PROGRAM Auto
VAR
	//////////////////////自动////////////////////////////////////////////
	//输入
	start AT%I* : BOOL;                        //启动按钮
	stop AT%I* : BOOL;                         //停止按钮
	//延时
	delayed_time: TON;                         //下限位延时功能块
	//其他
	state:INT;                                 //状态
	R_TRIG: R_TRIG;                            //检测下限位上升沿信号
	cycle_count:INT;                           //计数
	//超时监控
	watch_timer :ARRAY[1..2]OF TON;//工作计时
	bErr: BOOL;//报错
	ierrorID: INT:=0;//报错代码
END_VAR

CASE state OF
	0://初始状态
	   solenoid_valve_up := FALSE;                                     //上行电磁阀松开
       solenoid_valve_down := FALSE;	                               //下行电磁阀松开
       cycle_count := 0;                                               // 重置循环次数
	   bErr :=FALSE;                                               //报错复位
	   ierrorID :=0;                                               //报错代码复位
	   IF start THEN
	      solenoid_valve_down := TRUE;                                 // 下行电磁阀吸合，气缸下行
          state := 1;                                              
	   END_IF
	1://下行阶段  
	  solenoid_valve_down := TRUE;
      IF limit_switch_down THEN                                      //到达下限位
         solenoid_valve_down := FALSE;                              //下行电磁阀松开
      END_IF;
		 delayed_time(IN:=limit_switch_down , PT:=T#3S , Q=> , ET=> );  // 启动3秒延时
      IF delayed_time.Q THEN
         solenoid_valve_up := TRUE;                                 // 上行电磁阀吸合
         state := 2;                                                                                                                   
      END_IF;
    2://上行阶段
	  solenoid_valve_up := TRUE;
	  R_TRIG(CLK:=limit_switch_UP , Q=> );
      IF R_TRIG.Q THEN
         cycle_count := cycle_count + 1;                              // 循环次数+1
         solenoid_valve_up := FALSE;                                  // 上行电磁阀松开
         state := 1;                                                  // 切换回下行状态（开始下一次循环）
      END_IF;
      IF cycle_count >= 3 THEN                                        //清洗次数达到3次回到初始位
         state := 0;
      END_IF; 
    3://按下停止按钮后强制上行到上限位
      IF limit_switch_UP THEN                                       
         solenoid_valve_up := FALSE;                                 // 松开上行电磁阀
         state := 0;                                                 // 回到初始状态（停止所有动作）
      END_IF;  
END_CASE

IF stop THEN                                                         //按下停止按钮
   solenoid_valve_up := TRUE;                                        //上行电磁阀吸合
   solenoid_valve_down := FALSE;                                     //下行电磁阀松开
   state:=3;
END_IF

///////////超时计时器////////////////////////////////////////////////////////////
watch_timer[1](IN:=solenoid_valve_down , PT:=T#8S , Q=> , ET=> );  //气缸下行计时
watch_timer[2](IN:=solenoid_valve_up , PT:=T#8S , Q=> , ET=> );    //气缸上行计时
//超时报错
IF watch_timer[1].Q  AND NOT limit_switch_down THEN     //下行计时器超时，还未到达下限位，报错，报错代码为1
   bErr :=TRUE;
   ierrorID :=1;//下行超时代码  
END_IF
IF watch_timer[2].Q  AND NOT limit_switch_UP THEN       //上行计时器超时，还未到达上限位，报错，报错代码为2
   bErr :=TRUE;
   ierrorID :=2;//上行超时代码
END_IF

END_PROGRAM
